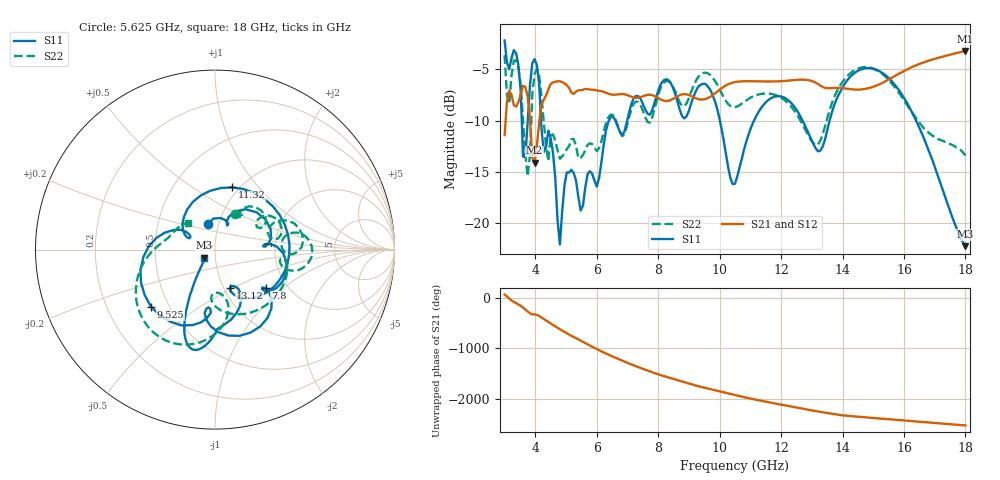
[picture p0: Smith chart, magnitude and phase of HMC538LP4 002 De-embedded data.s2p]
! Chelmsford, MA 01824
! http://www.hittite.com
! Tel: 978-250-3343
! Fax: 978-250-3373
! Device  :  HMC538LP4
! Description:  600 Analog Phase Shifter
! Frequency  :  6.0 GHz - 15.0 GHz
! Package  :  LP4  - 4x4 mm Quad Flatpack No-Lead (QFN) Plastic Package: 24 pin
! Ports  :  2 RF, 1 DC
!  Pin  3  = Rfin  = Port 1
!  Pin  16  = Rfout = Port 2
!  pin  21  = vCTL
! Voltages:  VCTL  = 0 to 5.0 Volts
! Currents :  Vb(V)  Vd(V)  Ib(mA)  Id(mA)
!  0.00  0.20  0.000000	0.485550
! Data:  The device was measured on evaluation board 111296-1.
!  Data was collected using a calibrated network analyzer.
!  The evaluation circuit board was modeled and simulated.This was use
!  to removed the evaluation board circuit from the measured data.
!  The reference plane is the center of the package pin.
! Misc:  Lot #
!Date Measured:  03 - 11 -2009
! Date:  03 - 17 -2009
! Note:
!  Hittite Microwave supplies this data as a sample of measured data at the
!  package pin for this package product.  Your particular data for this product
!  may vary.
!  Data was taken at 25 degrees C.
!  Hittite Microwave reserves the right to change this data at anytime.
# MHz S MA R 50
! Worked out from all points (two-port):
!   201 points, 3 GHz to 18 GHz, reference 50 ohm
!   highest |S21| = -3.20 dB at 18 GHz (marker M1); lowest = -14.1 dB at 3.975 GHz (marker M2)
!   |S21| within 3 dB of the highest: 10.61 GHz to 13.05 GHz (2.44 GHz wide, 20.6 % of centre); 15.38 GHz to end of sweep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
!   lowest |S11| = -22.3 dB at 18 GHz (marker M3), VSWR 1.17, Z = 44 - j4.05 ohm
!   |S11| at or under -10 dB: 4.187 GHz to 6.397 GHz (2.211 GHz wide, 41.8 % of centre); 10.01 GHz to 11.12 GHz (1.113 GHz wide, 10.5 % of centre); 16.39 GHz to end of sweep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
!   |S22| runs from -15.5 to -3.6 dB; largest |S21 - S12| = 0.002
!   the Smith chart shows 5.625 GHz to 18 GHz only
!   S11 on the Smith chart (normalised r, x): 5.625 GHz: 0.89, +0.26; 7.8 GHz: 1.56, -0.76; 9.525 GHz: 0.40, -0.33; 11.32 GHz: 0.93, +0.74; 13.12 GHz: 1.07, -0.49; 18 GHz: 0.88, -0.08
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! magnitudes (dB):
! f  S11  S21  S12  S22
! 3 GHz  -2.2  -11.4  -11.4  -3.6
! 3.15 GHz  -5.0  -7.1  -7.1  -8.3
! 3.45 GHz  -4.6  -8.2  -8.2  -4.9
! 3.6 GHz  -13.5  -6.6  -6.6  -10.0
! 3.75 GHz  -10.2  -7.6  -7.6  -15.5
! 3.975 GHz  -4.0  -14.1  -14.1  -5.4
! 4.275 GHz  -13.1  -8.0  -8.0  -10.2
! 4.575 GHz  -13.2  -6.3  -6.3  -11.4
! 4.8 GHz  -22.1  -6.2  -6.2  -13.7
! 5.025 GHz  -15.1  -6.5  -6.6  -12.8
! 5.55 GHz  -18.3  -7.0  -7.0  -13.4
! 5.625 GHz  -16.6  -6.9  -6.9  -12.9
! 7.8 GHz  -9.0  -7.5  -7.5  -9.7
! 8.025 GHz  -6.9  -7.9  -7.9  -7.3
! 9.525 GHz  -6.4  -7.9  -7.9  -5.3
! 10.5 GHz  -16.2  -6.2  -6.2  -8.7
! 11.32 GHz  -8.9  -6.2  -6.2  -7.4
! 13.05 GHz  -12.3  -6.2  -6.2  -12.2
! 13.12 GHz  -12.7  -6.3  -6.3  -12.4
! 14.25 GHz  -5.7  -6.9  -6.9  -5.4
! 15.53 GHz  -5.9  -5.9  -6.0  -6.1
! 18 GHz  -22.3  -3.2  -3.2  -13.4
